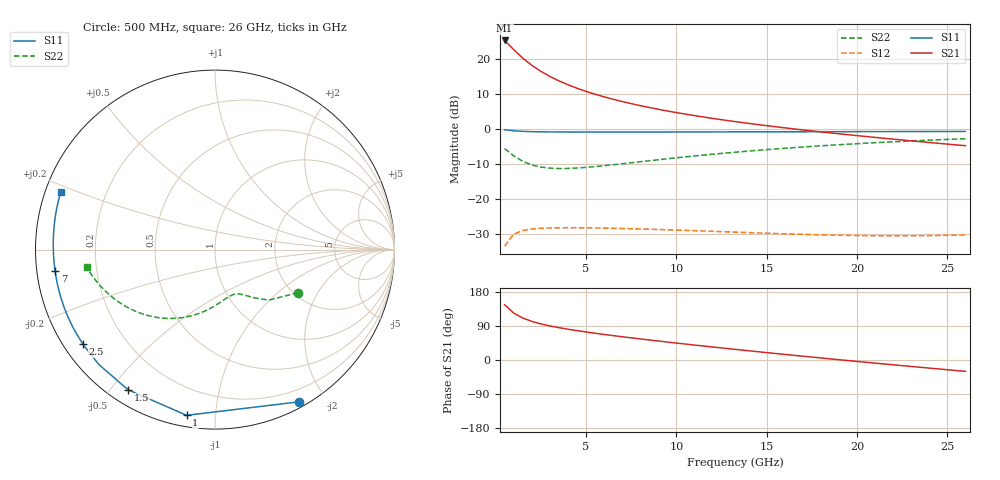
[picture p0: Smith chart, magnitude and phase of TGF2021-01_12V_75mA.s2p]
!TGF2021-01
!Unmatched Modeled S-parameters for 1mm pHEMT
!Vd = 12V Idq = 75mA
# GHz  S  DB  R  50
!Frequency s11	s11 ang	s21	s21 ang	s12	s12 ang	s22	s22 ang
!(GHz)	dB	deg	dB	deg	dB	deg	dB	deg
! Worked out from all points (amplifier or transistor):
!   52 points, 500 MHz to 26 GHz, reference 50 ohm
!   highest |S21| = 25.3 dB at 500 MHz (marker M1)
!   |S21| within 3 dB of that: start of sweep to 1.08 GHz
!   unconditionally stable (mu >= 1): 9.457 GHz to end of sweep
!   at 4.5 GHz: K = 0.48, MSG = 20.0 dB, |S12| = -28.3 dB
!   at 13.5 GHz: K = 1.38, MAG = 12.1 dB, |S12| = -29.6 dB
!   at 26 GHz: K = 1.55, MAG = 8.4 dB, |S12| = -30.3 dB
!   S11 on the Smith chart (normalised r, x): 500 MHz: 0.06, -1.70; 1 GHz: 0.06, -0.84; 1.5 GHz: 0.06, -0.55; 2.5 GHz: 0.05, -0.32; 7 GHz: 0.05, -0.07; 26 GHz: 0.04, +0.18
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0.5  -0.27 -61.0  25.26 145.9  -33.56 57.9  -5.66 -27.4
1  -0.57 -99.7  22.65 124.0  -30.16 38.2  -7.70 -43.1
1.5  -0.73 -121.8  20.21 110.8  -29.09 27.1  -9.30 -51.4
2  -0.82 -135.4  18.16 102.0  -28.66 20.3  -10.34 -56.6
2.5  -0.86 -144.4  16.44 95.3  -28.45 15.8  -10.94 -60.7
3  -0.89 -150.8  14.98 90.0  -28.35 12.5  -11.25 -64.3
3.5  -0.90 -155.6  13.72 85.4  -28.31 10.0  -11.36 -67.9
4  -0.91 -159.4  12.60 81.3  -28.30 8.1  -11.34 -71.4
4.5  -0.92 -162.5  11.61 77.5  -28.30 6.4  -11.22 -74.8
5  -0.92 -165.1  10.71 74.0  -28.33 5.1  -11.04 -78.2
5.5  -0.93 -167.3  9.89 70.7  -28.36 3.9  -10.81 -81.5
6  -0.93 -169.2  9.14 67.5  -28.40 2.9  -10.56 -84.8
7  -0.93 -172.4  7.80 61.4  -28.51 1.3  -10.01 -91.1
8  -0.92 -175.1  6.63 55.7  -28.64 0.0  -9.43 -97.0
9  -0.92 -177.3  5.58 50.1  -28.79 -0.9  -8.86 -102.7
11  -0.90 178.8  3.78 39.5  -29.13 -2.0  -7.78 -113.2
13.5  -0.88 174.9  1.89 26.9  -29.59 -2.0  -6.59 -125.1
15.5  -0.86 172.0  0.58 17.1  -29.95 -1.0  -5.76 -133.9
17.5  -0.84 169.4  -0.60 7.7  -30.26 0.8  -5.04 -142.1
19.5  -0.82 167.0  -1.69 -1.5  -30.48 3.4  -4.41 -149.8
22  -0.80 164.0  -2.96 -12.7  -30.59 7.3  -3.72 -158.9
26  -0.76 159.5  -4.84 -29.9  -30.35 13.6  -2.83 -172.4
